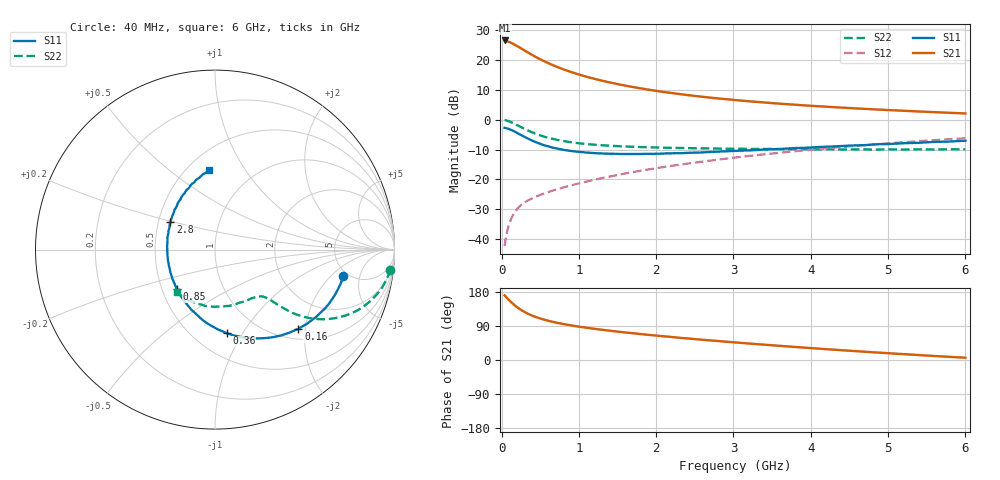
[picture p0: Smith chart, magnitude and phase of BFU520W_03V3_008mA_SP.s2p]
! Filename:  P:\Prog\Test\Noise\ATS_data\Testdata_Net\Run2\BFU520W_APM2013_06_A05_03p3V_008mA_SP_CM01_D.s2p
! Date/Time: Tue 26/Mar/2013 18:01:38
! BFU520W_APM2013_06_A05_03p3V_1to20mA_SP_CM01_Bias5_R.s2p
! MDIF S-parameter v. bias file
! BFU520W_APM2013_06_A05_03p3V_1to20mA_SP_CM01
! Date/time Tue Mar 19 16:47:37 2013
! VAR V_out= 3.3000
! VAR I_out= 7.9950
! VAR V_in= 0.8434
! VAR I_in= 0.0925
! Device data file deembeded for feedlines and parallel
! Original file: \Run2\BFU520W_APM2013_06_A05_03p3V_008mA_SP_CM01_R.s2p
! Feed-files: PR019V01_070313_Feed1.s2p, PR019V01_070313_Feed2.s2p
! Parallel-file: PR019V01_070313_Par.s2p
# MHz S MA R 50
!  Freq-MHz  S11-mag  S11-arg  S21-mag  S21-arg  S12-mag  S12-arg  S22-mag  S22-arg
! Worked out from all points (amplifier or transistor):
!   98 points, 40 MHz to 6 GHz, reference 50 ohm
!   highest |S21| = 26.5 dB at 40 MHz (marker M1)
!   |S21| within 3 dB of that: start of sweep to 275.2 MHz
!   unconditionally stable (mu >= 1): 1.484 GHz to 2.798 GHz
!   at 300 MHz: K = 0.46, MSG = 25.4 dB, |S12| = -27.7 dB
!   at 1.6 GHz: K = 1.01, MAG = 14.1 dB, |S12| = -18.0 dB
!   at 6 GHz: K = 0.87, MSG = 4.2 dB, |S12| = -6.2 dB
!   S11 on the Smith chart (normalised r, x): 40 MHz: 4.53, -2.87; 160 MHz: 1.22, -1.83; 360 MHz: 0.71, -0.85; 850 MHz: 0.60, -0.29; 2.8 GHz: 0.58, +0.19; 6 GHz: 0.64, +0.70
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40  0.7304 -11.7  21.12 170.4  0.007646 84.0  0.9829 -6.5
50  0.7266 -14.5  21.07 168.2  0.009447 83.0  0.9786 -8.1
80  0.7088 -23.0  20.36 161.6  0.01472 78.9  0.9548 -12.8
100  0.6941 -28.3  19.87 157.5  0.01803 76.6  0.9342 -15.6
120  0.6766 -33.7  19.44 153.5  0.02114 74.4  0.9126 -18.3
160  0.6404 -43.5  18.24 146.3  0.02683 70.4  0.8645 -23.0
200  0.6027 -52.6  17.06 139.8  0.03165 67.4  0.8134 -26.9
240  0.5641 -61.0  15.95 133.9  0.03583 65.2  0.7651 -30.1
300  0.5136 -72.3  14.32 126.6  0.04121 62.8  0.6989 -33.7
360  0.4699 -82.1  12.87 120.5  0.04581 61.3  0.643 -36.2
440  0.4225 -93.4  11.25 113.8  0.05132 60.4  0.5827 -38.4
550  0.3732 -106.6  9.517 106.5  0.05804 60.3  0.5196 -40.1
700  0.3321 -121.4  7.801 99.0  0.06724 61.0  0.4644 -41.4
850  0.3057 -133.7  6.588 93.1  0.07641 62.0  0.4279 -42.0
1050  0.2854 -147.0  5.451 86.6  0.08894 63.3  0.3966 -43.0
1500  0.2672 -170.3  3.936 74.9  0.1188 64.8  0.3608 -46.3
2050  0.2692 169.4  2.964 63.5  0.1575 64.6  0.3414 -52.3
2800  0.2919 148.4  2.263 50.0  0.2141 62.2  0.3279 -63.8
3100  0.3032 141.4  2.082 45.1  0.2384 60.8  0.3257 -68.8
4100  0.3484 122.4  1.677 30.0  0.3226 54.5  0.3175 -88.2
5200  0.4031 105.0  1.408 15.4  0.4195 45.4  0.3157 -112.5
6000  0.4443 94.0  1.27 6.0  0.4879 37.8  0.318 -132.3
